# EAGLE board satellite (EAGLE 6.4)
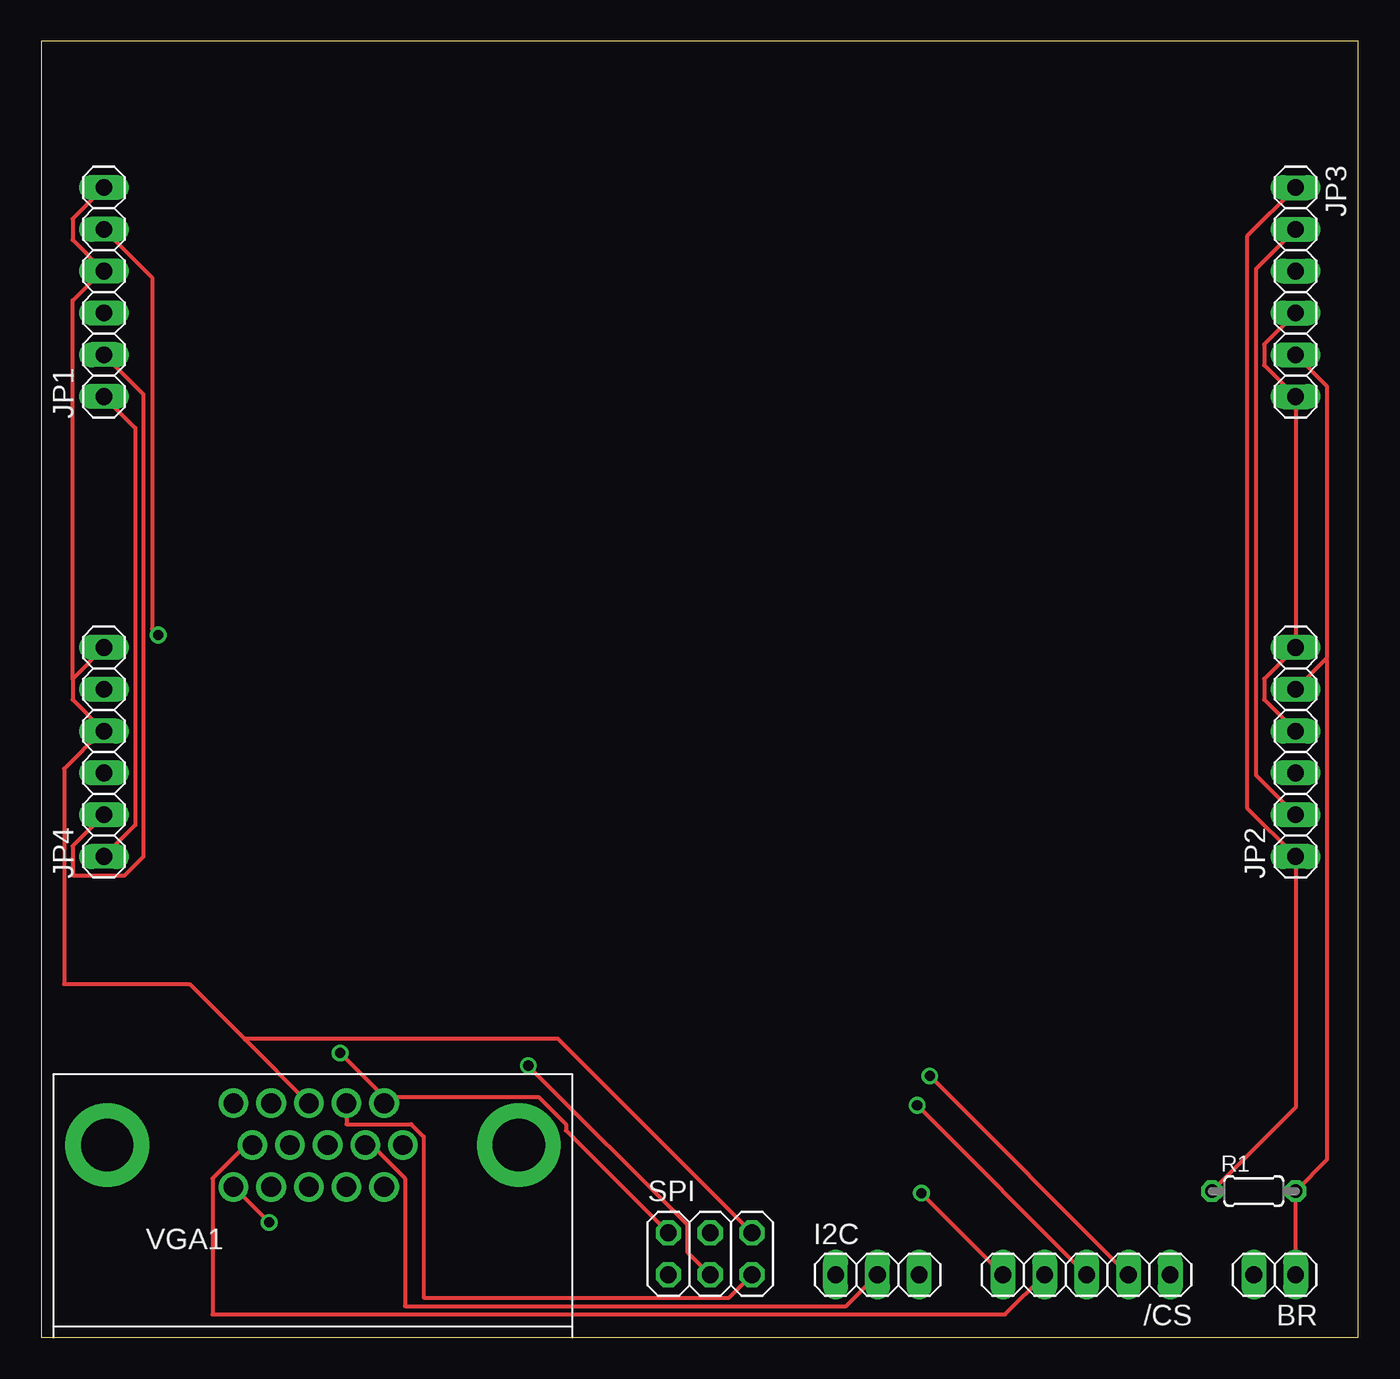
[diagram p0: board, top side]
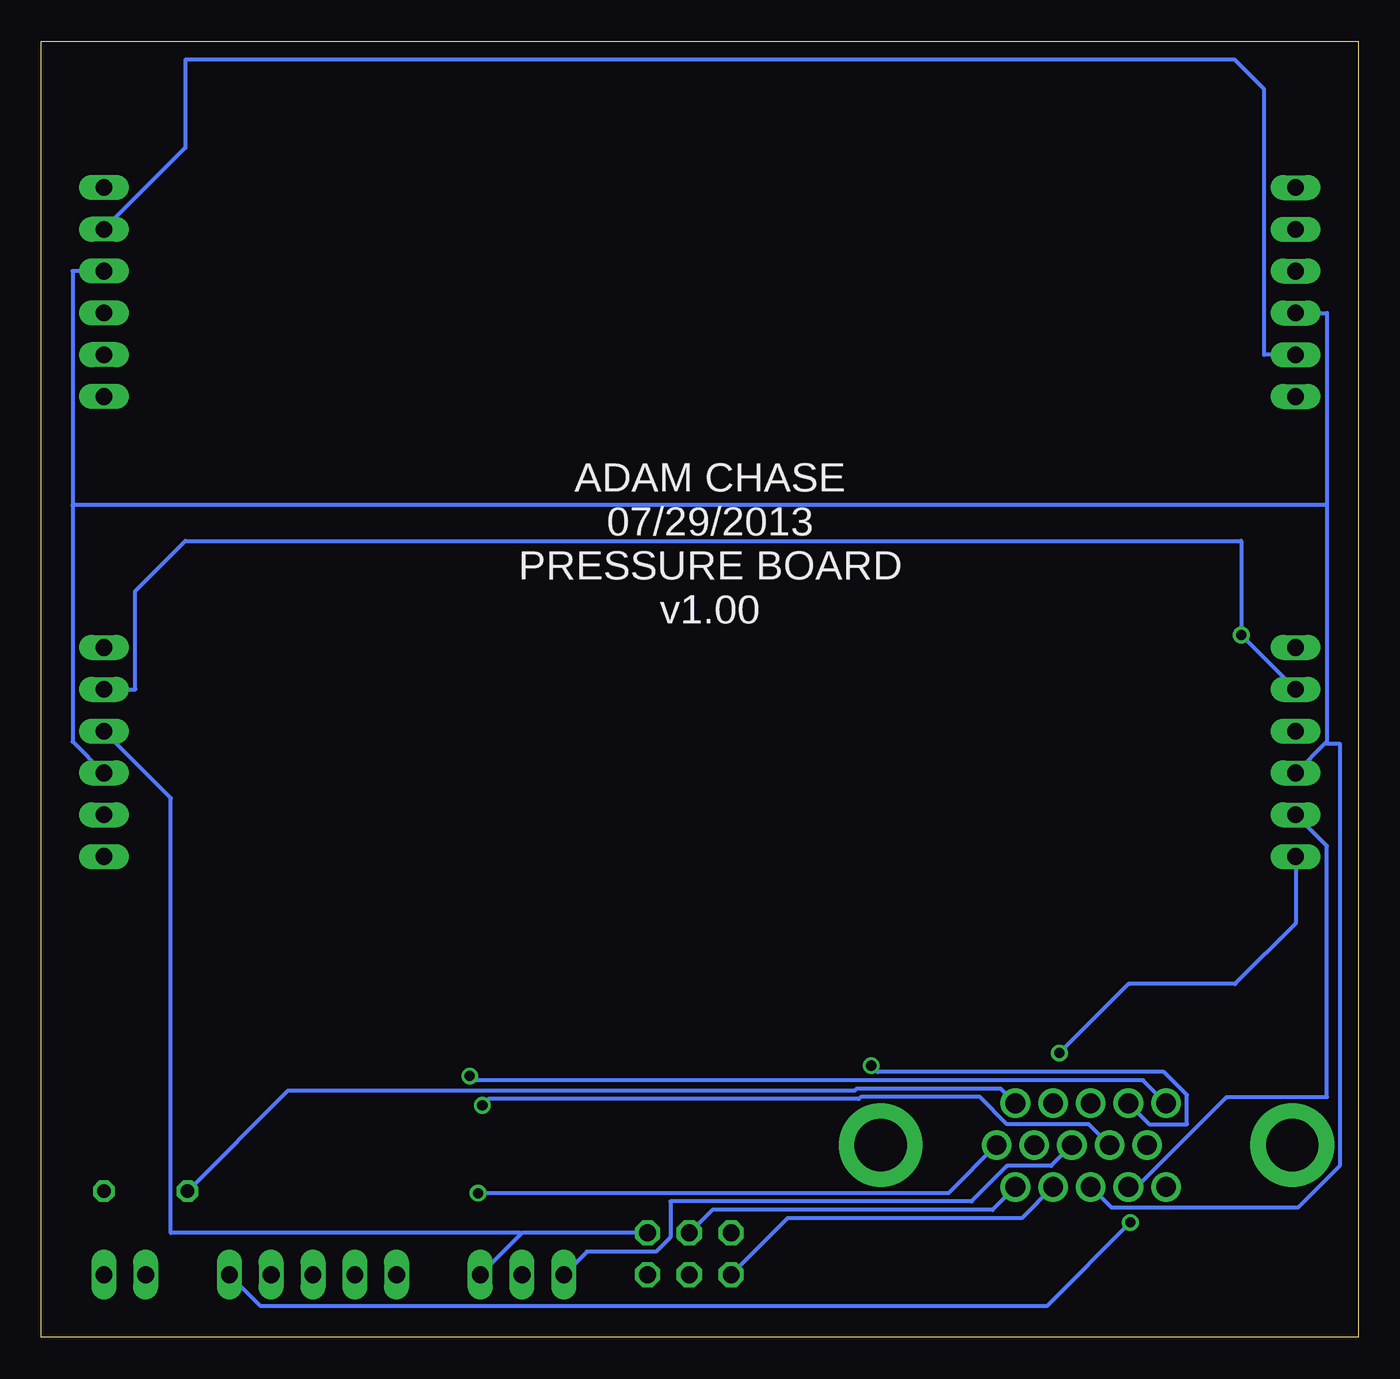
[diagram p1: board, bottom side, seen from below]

Size 80.01 x 78.74 mm. Coordinates in mm from the lower left corner, seen from the top.
Outline: 0,0 80.01,0 80.01,78.74 0,78.74 0,0
Copper layers (1*16): Top 0.035mm / dielectric 1.5mm / Bottom 0.035mm
Design rules "default": minimum track width 10mil, minimum drill 24mil, track to track 8mil, track to pad 8mil, pad to pad 8mil, via to via 8mil, smd to smd 8mil, copper to edge 40mil, drill to drill 8mil, minimum pad ring 10mil, minimum via ring 8mil, stop-mask expansion 4mil, vias tented up to drill 0mil, thermal gap 10mil
tRestrict: area 7.6,50.8 to 36.8,77.5; area 41.9,50.8 to 71.1,77.5; area 7.6,21.6 to 36.8,48.3; area 41.9,21.6 to 71.1,48.3
bRestrict: area 7.6,50.8 to 36.8,77.5; area 41.9,50.8 to 71.1,77.5; area 7.6,21.6 to 36.8,48.3; area 41.9,21.6 to 71.1,48.3

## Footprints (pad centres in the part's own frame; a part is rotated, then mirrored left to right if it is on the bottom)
1X05 = drill 1.016 long: 1 -5.08,0; 2 -2.54,0; 3 0,0; 4 2.54,0; 5 5.08,0
1X02 = drill 1.016 long: 1 -1.27,0; 2 1.27,0
1X03 = drill 1.016 long: 1 -2.54,0; 2 0,0; 3 2.54,0
1X06 = drill 1.016 long: 1 -6.35,0; 2 -3.81,0; 3 -1.27,0; 4 1.27,0; 5 3.81,0; 6 6.35,0
0204/5 = drill 0.813 octagon: 1 -2.54,0; 2 2.54,0
2X03 = drill 1.016 octagon: 1 -2.54,-1.27; 2 -2.54,1.27; 3 0,-1.27; 4 0,1.27; 5 2.54,-1.27; 6 2.54,1.27
DB-15-F90+SHIELD-SMALL_PADS = drill 1.2 pad 1.524: 1 4.318,14.224; 2 2.032,14.224; 3 -0.254,14.224; 4 -2.54,14.224; 5 -4.826,14.224; 6 5.461,11.684; 7 3.175,11.684; 8 0.889,11.684; 9 -1.397,11.684; 10 -3.683,11.684; 11 4.318,9.144; 12 2.032,9.144; 13 -0.254,9.144; 14 -2.54,9.144; 15 -4.826,9.144 | drill 3.175 pad 5.08: SHIELD@1 -12.497,11.684; SHIELD@2 12.497,11.684

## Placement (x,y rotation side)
/CS  [1X05]  63.5,3.81 180 top
BR  [1X02]  74.93,3.81 180 top
I2C  [1X03]  50.8,3.81 0 top
JP1  [1X06]  3.81,63.5 90 top
JP2  [1X06]  76.2,35.56 90 top
JP3  [1X06]  76.2,63.5 270 top
JP4  [1X06]  3.81,35.56 90 top
R1  4.7K  [0204/5]  73.66,8.89 0 top
SPI  [2X03]  40.64,5.08 0 top
VGA1  VGA-F90S  [DB-15-F90+SHIELD-SMALL_PADS]  16.51,0 0 top

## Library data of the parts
/CS BR I2C JP1-JP4 SPI = pinhead
R1 = rcl
VGA1 = VideoConnectors

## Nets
5V: JP1.1 JP2.1 JP3.1 JP4.1 R1.1 SPI.2 VGA1.1
33V: SPI.5 VGA1.2
BR: BR.1 JP1.5 JP2.5 JP3.5 JP4.5 R1.2
GND: I2C.3 JP1.4 JP1.6 JP2.4 JP2.6 JP3.4 JP3.6 JP4.4 JP4.6 SPI.6 VGA1.3
GPIO1: /CS.1 VGA1.15
GPIO2: /CS.2 VGA1.5
GPIO3: /CS.3 VGA1.9
GPIO4: /CS.4 VGA1.10
GPIO5: /CS.5 VGA1.6
MISO: SPI.1 VGA1.12
MOSI: SPI.4 VGA1.11
RX: JP1.3 JP2.3 JP3.3 JP4.3 VGA1.13
SCL: I2C.2 VGA1.7
SCLK: SPI.3 VGA1.4
SDA: I2C.1 VGA1.8
TX: JP1.2 JP2.2 JP3.2 JP4.2 VGA1.14

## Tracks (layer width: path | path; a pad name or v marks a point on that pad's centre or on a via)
5V  (via drill 0.61)
  Top 0.254: R1.1 76.2,13.97 JP2.1 73.28,32.13 73.28,66.93 JP3.1 | SPI.2 31.88,12.57 31.88,12.95 30.23,14.61 20.83,14.61 | JP4.1 5.71,31.11 5.71,55.24 JP1.1 | v18.16,17.27 20.83,14.61 | 20.83,14.61 VGA1.1
  Bottom 0.254: v18.16,17.27 13.97,21.46 7.49,21.46 3.81,25.15 JP4.1 | R1.1 65.02,14.99 30.61,14.99 30.48,15.11 21.72,15.11 VGA1.1
33V
  Top 0.254: SPI.5 41.78,2.41 23.24,2.41 23.24,12.19 22.48,12.95 18.54,12.95 VGA1.2
BR  (via drill 0.61)
  Top 0.254: v7.11,42.67 6.73,43.05 6.73,64.39 JP1.5 | BR.1 R1.2 78.11,10.79 78.11,41.15 78.04,41.21 | 78.04,41.21 78.11,41.27 78.11,57.78 JP3.5 | 78.04,41.21 JP2.5
  Bottom 0.254: JP4.5 v7.11,42.67 7.11,48.39 71.25,48.39 74.3,45.34 74.3,39.37 JP2.5
GND
  Top 0.254: JP2.4 74.3,38.73 74.3,40.01 JP2.6 JP3.6 74.3,59.05 74.3,60.33 JP3.4 | JP1.6 1.91,67.94 1.91,66.67 JP1.4 3.68,64.77 1.91,62.99 1.91,40.13 1.97,40.07 | JP4.6 1.97,40.07 | 1.97,40.07 1.91,40.01 1.91,38.73 JP4.4 3.68,36.83 1.4,34.54 1.4,21.46 9.02,21.46 12.38,18.1 | 12.38,18.1 VGA1.3 | SPI.6 31.37,18.16 12.45,18.16 12.38,18.1
  Bottom 0.254: 50.86,6.29 50.8,6.35 SPI.6 | 50.86,6.29 I2C.3 | JP2.4 72.14,32.77 72.14,6.35 50.93,6.35 50.86,6.29
GPIO1  (via drill 0.61)
  Top 0.254: VGA1.15 v13.84,6.99
  Bottom 0.254: /CS.1 66.67,1.91 18.92,1.91 v13.84,6.99
GPIO2  (via drill 0.61)
  Top 0.254: v53.98,15.88 /CS.2
  Bottom 0.254: v53.98,15.88 53.72,15.62 13.08,15.62 VGA1.5
GPIO3  (via drill 0.61)
  Top 0.254: v53.21,14.1 /CS.3
  Bottom 0.254: v53.21,14.1 52.83,14.48 30.35,14.48 30.23,14.61 22.99,14.61 21.34,12.95 16.38,12.95 VGA1.9
GPIO4
  Top 0.254: /CS.4 58.55,1.4 10.41,1.4 10.41,9.65 12.45,11.68 VGA1.10
GPIO5  (via drill 0.61)
  Top 0.254: v53.47,8.76 /CS.5
  Bottom 0.254: v53.47,8.76 24.89,8.76 VGA1.6
MISO
  Bottom 0.254: SPI.1 34.67,7.24 20.45,7.24 VGA1.12
MOSI
  Bottom 0.254: SPI.4 39.24,7.75 22.23,7.75 VGA1.11
RX
  Bottom 0.254: JP2.3 78.11,36.2 78.11,50.55 | 78.11,50.55 78.11,64.77 JP3.3 | 1.97,36.13 1.91,36.2 1.91,50.55 | 1.97,36.13 JP4.3 | 1.91,50.55 1.91,62.23 JP1.3 | VGA1.13 14.99,7.87 3.68,7.87 1.14,10.41 1.14,36.07 1.91,36.07 1.97,36.13 | 1.91,50.55 78.11,50.55
SCL
  Top 0.254: I2C.2 48.9,1.91 22.1,1.91 22.1,9.65 20.07,11.68 VGA1.7
SCLK  (via drill 0.61)
  Top 0.254: SPI.3 39.24,5.21 39.24,6.86 v29.59,16.51
  Bottom 0.254: v29.59,16.51 29.21,16.13 11.81,16.13 10.41,14.73 10.41,12.95 12.7,12.95 VGA1.4
SDA
  Bottom 0.254: I2C.1 46.86,5.21 42.67,5.21 41.78,6.1 41.78,8.26 23.5,8.26 21.34,10.41 18.67,10.41 VGA1.8
TX
  Top 0.254: JP2.2 73.79,34.16 73.79,64.9 JP3.2 | JP1.2 6.22,57.28 6.22,29.21 5.08,28.07 1.91,28.07 1.91,29.84 JP4.2
  Bottom 0.254: JP4.2 1.91,29.84 1.91,14.61 8,14.61 13.46,9.14 VGA1.14 | JP3.2 71.25,72.26 71.25,77.6 7.49,77.6 5.71,75.82 5.71,59.69 JP1.2

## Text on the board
bPlace: ADAM CHASE / 07/29/2013 / PRESSURE BOARD / v1.00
